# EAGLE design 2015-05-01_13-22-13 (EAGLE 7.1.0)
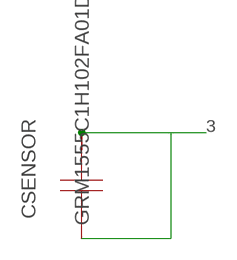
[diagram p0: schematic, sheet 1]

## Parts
CSENSOR  GRM1555C1H102FA01D  [0402]

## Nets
3: CSENSOR.1 CSENSOR.2

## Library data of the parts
CSENSOR = ultra-librarian:GRM1555C1H102FA01D; CAP: 1.0E-9; DATASHEETURL: http://search.murata.co.jp/Ceramy/image/img/A01X/G101/ENG/GRM1555C1H102FA01%2D01.pdf; ESR: 0.0; IRMS: 0.0; MANUFACTURER_PART_NUMBER: GRM1555C1H102FA01D; VDC: 50.0; VENDOR: MuRata

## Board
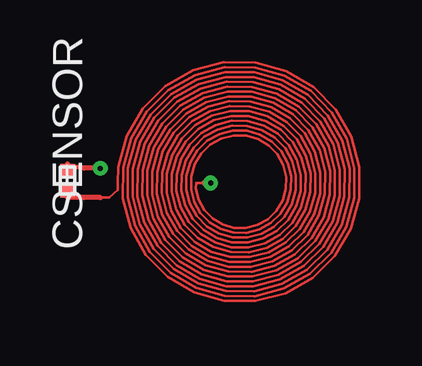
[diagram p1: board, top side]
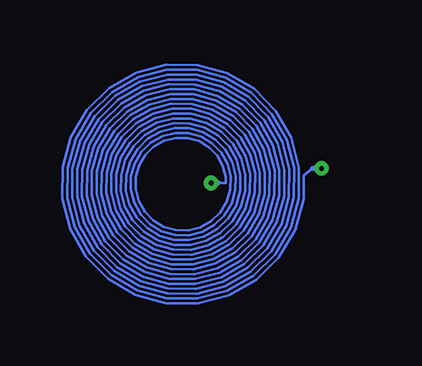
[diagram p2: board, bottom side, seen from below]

No outline drawn. Coordinates in mm, seen from the top.
Copper layers ((1*2)+(15*16)): TOP 0.035mm / dielectric 1.5mm / INTERNAL1 0.035mm / dielectric 0.15mm / layer 15 0.035mm / dielectric 0.2mm / BOTTOM 0.035mm
Design rules "custom": minimum track width 10mil, minimum drill 0.6mm, track to track 8mil, track to pad 8mil, pad to pad 8mil, via to via 8mil, smd to smd 8mil, copper to edge 40mil, drill to drill 8mil, minimum pad ring 10mil, minimum via ring 8mil, stop-mask expansion 4mil, vias tented up to drill 0mil, thermal gap 10mil

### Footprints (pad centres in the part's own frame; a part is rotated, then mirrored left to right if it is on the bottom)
0402 = smd 0.559 x 0.61: 1 -0.419,0; 2 0.419,0

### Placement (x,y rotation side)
CSENSOR  [0402]  6.73,8.2 90 top

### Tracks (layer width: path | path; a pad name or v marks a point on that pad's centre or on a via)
3  (via drill 0.2 pad 0.61)
  TOP 0.102: 12.4,8.11 12.1,8.11 12.09,7.87 12.21,7.4 12.44,6.97 12.78,6.62 13.2,6.37 13.67,6.24 14.17,6.23 14.65,6.35 15.08,6.59 15.44,6.94 15.7,7.37 15.84,7.86 15.85,8.36 15.73,8.86 15.48,9.3 15.12,9.67 14.68,9.94 14.18,10.08 13.66,10.09 13.15,9.96 12.69,9.71 12.31,9.34 12.04,8.88 11.9,8.37 11.89,7.84 12.02,7.32 12.28,6.85 12.66,6.46 13.12,6.18 13.65,6.03 14.19,6.03 14.73,6.16 15.21,6.43 15.61,6.81 15.89,7.29 16.04,7.83 16.05,8.39 15.91,8.93 15.64,9.43 15.24,9.84 14.76,10.13 14.21,10.28 13.63,10.29 13.07,10.15 12.57,9.87 12.15,9.46 11.85,8.96 11.69,8.4 11.68,7.81 11.83,7.24 12.12,6.72 12.53,6.3 13.04,5.99 13.62,5.83 14.22,5.82 14.8,5.97 15.33,6.26 15.77,6.69 16.08,7.21 16.25,7.8 16.26,8.41 16.1,9.01 15.8,9.55 15.37,10 14.83,10.32 14.23,10.49 13.61,10.49 12.99,10.34 12.44,10.03 11.99,9.59 11.66,9.04 11.49,8.43 11.48,7.79 11.64,7.16 11.96,6.6 12.41,6.14 12.96,5.8 13.59,5.63 14.25,5.62 14.88,5.78 15.46,6.1 15.93,6.56 16.27,7.13 16.45,7.77 16.46,8.44 16.29,9.09 15.96,9.68 15.49,10.16 14.91,10.51 14.26,10.69 13.58,10.7 12.92,10.53 12.32,10.19 11.83,9.71 11.47,9.12 11.29,8.45 11.28,7.76 11.45,7.08 11.79,6.48 12.28,5.97 12.89,5.62 13.57,5.42 14.27,5.42 14.96,5.59 15.58,5.94 16.09,6.44 16.46,7.06 16.65,7.75 16.66,8.47 16.48,9.17 16.13,9.8 15.62,10.32 14.99,10.7 14.29,10.89 13.55,10.9 12.84,10.72 12.19,10.36 11.66,9.84 11.28,9.2 11.08,8.48 11.07,7.73 11.26,7.01 11.63,6.35 12.16,5.81 12.81,5.43 13.54,5.22 14.3,5.21 15.04,5.4 15.71,5.78 16.26,6.31 16.65,6.98 16.86,7.72 16.86,8.49 16.67,9.25 16.29,9.93 15.74,10.48 15.07,10.88 14.31,11.1 13.53,11.1 12.76,10.91 12.07,10.52 11.5,9.96 11.1,9.28 10.88,8.51 10.87,7.71 11.07,6.93 11.47,6.23 12.03,5.65 12.73,5.24 13.51,5.02 14.33,5.01 15.12,5.21 15.83,5.62 16.42,6.19 16.84,6.9 17.06,7.69 17.07,8.52 16.86,9.33 16.45,10.05 15.87,10.65 15.15,11.07 14.34,11.3 13.5,11.31 12.68,11.1 11.94,10.68 11.34,10.09 10.91,9.36 10.68,8.53 10.67,7.68 10.88,6.85 11.3,6.1 11.91,5.49 12.65,5.05 13.49,4.82 14.35,4.81 15.2,5.02 15.96,5.45 16.58,6.07 17.03,6.82 17.26,7.67 17.27,8.55 17.05,9.4 16.61,10.18 15.99,10.81 15.23,11.26 14.37,11.5 13.47,11.51 12.6,11.29 11.82,10.84 11.18,10.21 10.72,9.43 10.47,8.56 10.46,7.65 10.69,6.77 11.14,5.98 11.78,5.32 12.57,4.86 13.46,4.61 14.38,4.6 15.28,4.83 16.08,5.29 16.74,5.94 17.22,6.74 17.47,7.64 17.48,8.58 17.24,9.48 16.78,10.3 16.12,10.97 15.3,11.45 14.39,11.71 13.44,11.71 12.52,11.48 11.69,11.01 11.01,10.34 10.53,9.51 10.27,8.59 10.26,7.63 10.5,6.69 10.98,5.85 11.66,5.16 12.49,4.67 13.43,4.41 14.41,4.4 15.35,4.64 16.21,5.13 16.91,5.82 17.41,6.66 17.67,7.61 17.68,8.6 17.43,9.56 16.94,10.43 16.24,11.14 15.38,11.64 14.42,11.91 13.42,11.92 12.45,11.66 11.57,11.17 10.85,10.46 10.34,9.59 10.07,8.62 10.06,7.6 10.31,6.61 10.82,5.73 11.53,5 12.42,4.48 13.4,4.21 14.43,4.2 15.43,4.46 16.33,4.96 17.07,5.69 17.59,6.58 17.87,7.59 17.88,8.63 17.62,9.64 17.1,10.55 16.37,11.3 15.46,11.83 14.45,12.11 13.39,12.12 12.37,11.86 11.45,11.33 10.69,10.59 10.15,9.67 9.86,8.64 9.86,7.57 10.12,6.54 10.65,5.6 11.41,4.84 12.34,4.29 13.38,4 14.46,3.99 15.51,4.27 16.46,4.8 17.23,5.57 17.79,6.51 18.08,7.56 18.08,8.66 17.81,9.72 17.27,10.68 16.49,11.46 15.54,12.02 14.47,12.31 13.36,12.32 12.29,12.04 11.32,11.49 10.53,10.71 9.96,9.75 9.66,8.67 9.65,7.55 9.94,6.46 10.49,5.48 11.28,4.67 12.26,4.1 13.35,3.8 14.49,3.79 15.59,4.08 16.58,4.64 17.39,5.44 17.97,6.43 18.28,7.53 18.29,8.68 18,9.8 17.43,10.8 16.62,11.62 15.62,12.21 14.5,12.52 13.34,12.53 12.21,12.23 11.2,11.66 10.36,10.84 9.77,9.83 9.46,8.7 9.45,7.52 9.75,6.38 10.33,5.35 11.16,4.51 12.18,3.91 13.32,3.6 14.51,3.59 15.67,3.89 16.7,4.48 17.56,5.32 18.16,6.35 18.48,7.51 18.49,8.71 18.19,9.88 17.59,10.93 16.74,11.79 15.7,12.4 14.53,12.72 13.31,12.73 12.13,12.42 11.07,11.82 10.2,10.96 9.58,9.9 9.26,8.72 9.25,7.49 9.56,6.3 10.17,5.23 11.03,4.35 12.1,3.72 13.3,3.39 14.54,3.38 15.75,3.7 16.83,4.31 17.72,5.19 18.35,6.27 18.69,7.48 18.69,8.74 18.38,9.95 17.75,11.05 16.87,11.95 15.78,12.59 14.55,12.93 13.28,12.93 12.05,12.61 10.95,11.98 10.04,11.09 9.39,9.98 9.05,8.75 9.04,7.47 9.37,6.22 10,5.1 10.91,4.18 12.02,3.53 13.27,3.19 14.57,3.18 15.82,3.51 16.95,4.15 17.88,5.07 18.54,6.19 18.89,7.45 18.9,8.76 18.57,10.03 17.92,11.18 16.99,12.11 15.85,12.78 14.58,13.13 13.26,13.14 11.97,12.8 10.82,12.14 9.88,11.21 9.2,10.06 8.85,8.78 8.84,8.11 8.84,7.8 8.47,7.5 8.11,7.5
  TOP 0.203: 12.4,8.11 v12.7,8.11 | v8.11,8.72 7.42,8.72 6.74,8.81 6.74,8.89 | 8.11,7.5 7.42,7.5 6.74,7.5
  BOTTOM 0.102: 12.4,8.11 12.1,8.11 12.09,8.35 12.21,8.82 12.44,9.24 12.78,9.59 13.2,9.84 13.67,9.98 14.17,9.99 14.65,9.87 15.08,9.62 15.44,9.28 15.7,8.85 15.84,8.36 15.85,7.85 15.73,7.36 15.48,6.91 15.12,6.54 14.68,6.28 14.18,6.13 13.66,6.13 13.15,6.25 12.69,6.51 12.31,6.88 12.04,7.33 11.9,7.84 11.89,8.38 12.02,8.89 12.28,9.37 12.66,9.75 13.12,10.03 13.65,10.18 14.19,10.19 14.73,10.06 15.21,9.79 15.61,9.4 15.89,8.93 16.04,8.39 16.05,7.83 15.91,7.28 15.64,6.79 15.24,6.38 14.76,6.09 14.21,5.93 13.63,5.92 13.07,6.07 12.57,6.35 12.15,6.75 11.85,7.25 11.69,7.82 11.68,8.4 11.83,8.97 12.12,9.49 12.53,9.92 13.04,10.22 13.62,10.38 14.22,10.39 14.8,10.24 15.33,9.95 15.77,9.53 16.08,9 16.25,8.41 16.26,7.8 16.1,7.2 15.8,6.66 15.37,6.22 14.83,5.9 14.23,5.73 13.61,5.72 12.99,5.88 12.44,6.18 11.99,6.63 11.66,7.17 11.49,7.79 11.48,8.43 11.64,9.05 11.96,9.62 12.41,10.08 12.96,10.41 13.59,10.59 14.25,10.6 14.88,10.44 15.46,10.11 15.93,9.65 16.27,9.08 16.45,8.44 16.46,7.77 16.29,7.12 15.96,6.54 15.49,6.05 14.91,5.71 14.26,5.53 13.58,5.52 12.92,5.69 12.32,6.02 11.83,6.5 11.47,7.09 11.29,7.76 11.28,8.46 11.45,9.13 11.79,9.74 12.28,10.24 12.89,10.6 13.57,10.79 14.27,10.8 14.96,10.62 15.58,10.28 16.09,9.78 16.46,9.16 16.65,8.47 16.66,7.75 16.48,7.05 16.13,6.41 15.62,5.89 14.99,5.52 14.29,5.32 13.55,5.31 12.84,5.5 12.19,5.86 11.66,6.38 11.28,7.02 11.08,7.73 11.07,8.48 11.26,9.21 11.63,9.87 12.16,10.4 12.81,10.79 13.54,10.99 14.3,11 15.04,10.81 15.71,10.44 16.26,9.9 16.65,9.24 16.86,8.49 16.86,7.72 16.67,6.97 16.29,6.29 15.74,5.73 15.07,5.33 14.31,5.12 13.53,5.11 12.76,5.31 12.07,5.7 11.5,6.25 11.1,6.94 10.88,7.71 10.87,8.51 11.07,9.29 11.47,9.99 12.03,10.57 12.73,10.98 13.51,11.2 14.33,11.21 15.12,11 15.83,10.6 16.42,10.03 16.84,9.32 17.06,8.52 17.07,7.69 16.86,6.89 16.45,6.16 15.87,5.57 15.15,5.14 14.34,4.92 13.5,4.91 12.68,5.12 11.94,5.53 11.34,6.13 10.91,6.86 10.68,7.68 10.67,8.54 10.88,9.37 11.3,10.11 11.91,10.73 12.65,11.17 13.49,11.4 14.35,11.41 15.2,11.19 15.96,10.76 16.58,10.15 17.03,9.39 17.26,8.55 17.27,7.67 17.05,6.81 16.61,6.04 15.99,5.41 15.23,4.95 14.37,4.71 13.47,4.71 12.6,4.93 11.82,5.37 11.18,6 10.72,6.78 10.47,7.65 10.46,8.56 10.69,9.44 11.14,10.24 11.78,10.89 12.57,11.36 13.46,11.6 14.38,11.61 15.28,11.38 16.08,10.93 16.74,10.28 17.22,9.47 17.47,8.57 17.48,7.64 17.24,6.73 16.78,5.91 16.12,5.24 15.3,4.76 14.39,4.51 13.44,4.5 12.52,4.74 11.69,5.21 11.01,5.88 10.53,6.7 10.27,7.63 10.26,8.59 10.5,9.52 10.98,10.36 11.66,11.05 12.49,11.55 13.43,11.81 14.41,11.82 15.35,11.57 16.21,11.09 16.91,10.4 17.41,9.55 17.67,8.6 17.68,7.61 17.43,6.65 16.94,5.79 16.24,5.08 15.38,4.57 14.42,4.31 13.42,4.3 12.45,4.55 11.57,5.05 10.85,5.75 10.34,6.62 10.07,7.6 10.06,8.62 10.31,9.6 10.82,10.49 11.53,11.22 12.42,11.74 13.4,12.01 14.43,12.02 15.43,11.76 16.33,11.25 17.07,10.53 17.59,9.63 17.87,8.63 17.88,7.59 17.62,6.58 17.1,5.67 16.37,4.92 15.46,4.38 14.45,4.1 13.39,4.09 12.37,4.36 11.45,4.88 10.69,5.63 10.15,6.55 9.86,7.57 9.86,8.64 10.12,9.68 10.65,10.61 11.41,11.38 12.34,11.93 13.38,12.21 14.46,12.22 15.51,11.95 16.46,11.41 17.23,10.65 17.79,9.71 18.08,8.65 18.08,7.56 17.81,6.5 17.27,5.54 16.49,4.75 15.54,4.2 14.47,3.9 13.36,3.89 12.29,4.17 11.32,4.72 10.53,5.5 9.96,6.47 9.66,7.55 9.65,8.67 9.94,9.76 10.49,10.74 11.28,11.54 12.26,12.12 13.35,12.42 14.49,12.43 15.59,12.14 16.58,11.58 17.39,10.77 17.97,9.79 18.28,8.68 18.29,7.53 18,6.42 17.43,5.42 16.62,4.59 15.62,4 14.5,3.7 13.34,3.69 12.21,3.98 11.2,4.56 10.36,5.38 9.77,6.39 9.46,7.52 9.45,8.7 9.75,9.84 10.33,10.86 11.16,11.71 12.18,12.3 13.32,12.62 14.51,12.63 15.67,12.33 16.7,11.74 17.56,10.9 18.16,9.87 18.48,8.71 18.49,7.51 18.19,6.34 17.59,5.29 16.74,4.43 15.7,3.82 14.53,3.49 13.31,3.48 12.13,3.79 11.07,4.39 10.2,5.25 9.58,6.31 9.26,7.49 9.25,8.72 9.56,9.91 10.17,10.99 11.03,11.87 12.1,12.49 13.3,12.82 14.54,12.83 15.75,12.52 16.83,11.9 17.72,11.02 18.35,9.94 18.69,8.73 18.69,7.48 18.38,6.26 17.75,5.17 16.87,4.27 15.78,3.63 14.55,3.29 13.28,3.28 12.05,3.6 10.95,4.23 10.04,5.13 9.39,6.23 9.05,7.47 9.04,8.75 9.37,9.99 10,11.11 10.91,12.03 12.02,12.68 13.27,13.03 14.57,13.04 15.82,12.71 16.95,12.06 17.88,11.15 18.54,10.02 18.89,8.76 18.9,7.45 18.57,6.18 17.92,5.04 16.99,4.1 15.85,3.44 14.58,3.09 13.26,3.08 11.97,3.41 10.82,4.07 9.88,5 9.2,6.15 8.85,7.44 8.84,8.11 8.84,8.41 8.47,8.72
  BOTTOM 0.203: 12.4,8.11 v12.7,8.11 | 8.47,8.72 v8.11,8.72

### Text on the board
Reference: Exported from WEBENCH Coil Designer Tool | ------------------------- | User Id - 1231471 | WEBENCH Design Information | -------------- | Coil Parameters | Layers = 2 | Design Id - 5227 | Exported on - 2015/05/01 13:22:11 | Version - 1.0 | Trace Spacing = 4.0 mils | Trace Width = 4.0 mils | Turns = 16 | Inner Diameter = 144 mils (Approx.) | Outer Diameter = 400 mils (Approx.)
